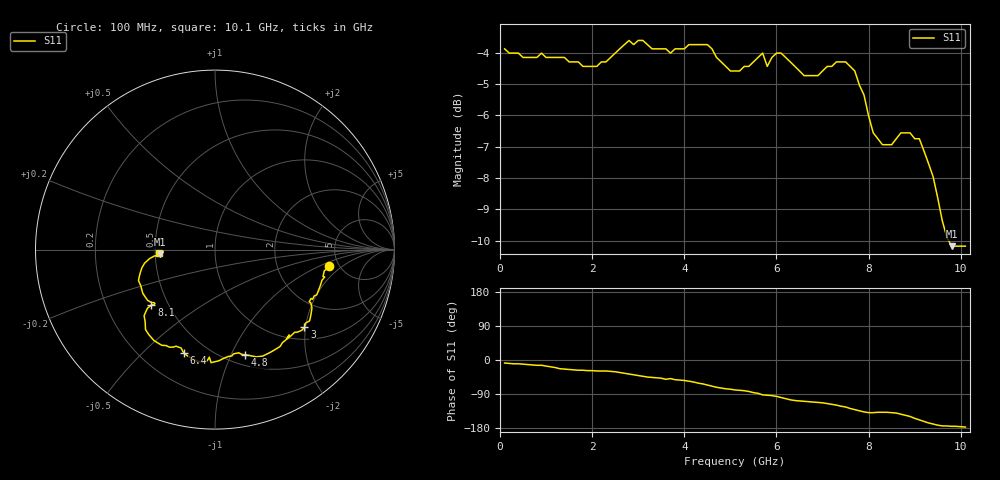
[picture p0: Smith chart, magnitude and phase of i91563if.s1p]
!	IAM-91563 IF Port S PARAMETERS
!	Vd = 3 V	LAST UPDATED 3-12-96
# ghz	s ma r	50
! Freq	IF(Mag)	IF(Ang)
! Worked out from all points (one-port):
!   101 points, 100 MHz to 10.1 GHz, reference 50 ohm
!   lowest |S11| = -10.2 dB at 9.8 GHz (marker M1), VSWR 1.90, Z = 26.4 - j1.58 ohm
!   |S11| at or under -10 dB: 9.737 GHz to end of sweep
!   S11 on the Smith chart (normalised r, x): 100 MHz: 4.16, -1.25; 3 GHz: 1.28, -1.97; 4.8 GHz: 0.61, -1.13; 6.4 GHz: 0.37, -0.67; 8.1 GHz: 0.40, -0.32; 10.1 GHz: 0.53, -0.02
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0.1  0.64 -8.0
0.9  0.63 -14.0
1.4  0.62 -24.0
2.3  0.61 -29.0
2.6  0.64 -33.0
3  0.66 -41.0
3.6  0.64 -51.0
3.7  0.63 -49.0
3.9  0.64 -53.0
4.5  0.65 -66.0
4.8  0.61 -74.0
5.1  0.59 -79.0
5.4  0.6 -83.0
5.7  0.63 -92.0
5.8  0.6 -93.0
6.1  0.63 -99.0
6.4  0.6 -107.0
7  0.59 -113.0
7.3  0.61 -119.0
7.6  0.6 -128.0
7.9  0.54 -137.0
8.1  0.47 -139.0
8.5  0.45 -139.0
8.9  0.47 -149.0
9.1  0.46 -158.0
9.5  0.37 -172.0
9.8  0.31 -175.0
10.1  0.31 -177.0
